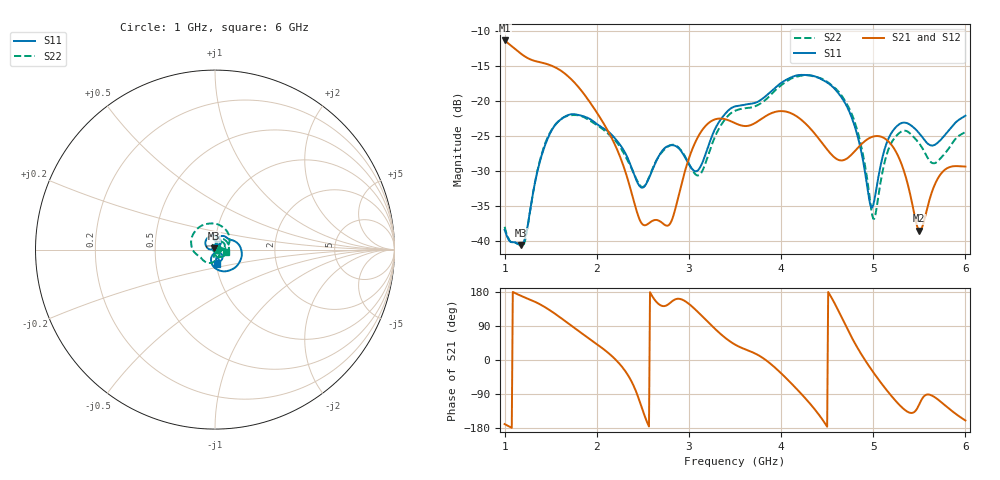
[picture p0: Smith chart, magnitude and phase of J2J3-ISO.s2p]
!Agilent Technologies,E8364B,MY43040528,A.07.50.67
!Agilent E8364B: A.07.50.67
!Date: Sunday, March 01, 2026 20:26:27
!Correction: S11(Full 2 Port(1,2))
!S21(Full 2 Port(1,2))
!S12(Full 2 Port(1,2))
!S22(Full 2 Port(1,2))
!S2P File: Measurements: S11, S21, S12, S22:
# Hz S  dB  R 50
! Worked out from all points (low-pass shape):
!   451 points, 1 GHz to 6 GHz, reference 50 ohm
!   highest |S21| = -11.35 dB at 1 GHz (marker M1); lowest = -38.5 dB at 5.5 GHz (marker M2)
!   |S21| within 3 dB of the highest: start of sweep to 1.349 GHz
!   lowest |S11| = -40.6 dB at 1.178 GHz (marker M3), VSWR 1.02, Z = 49.4 + j0.698 ohm
!   |S11| at or under -10 dB: start of sweep to end of sweep
!   |S22| runs from -40.7 to -16.3 dB; largest |S21 - S12| = 0.00066
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1e9  -38.38 74.1  -11.35 -169.1  -11.37 -169.1  -37.95 16.8
1.177778e9  -40.56 131.1  -13.24 169.3  -13.26 169.2  -40.68 67.7
1.477778e9  -25.04 155.8  -14.79 133.3  -14.80 133.3  -24.88 86.5
1.844444e9  -22.13 91.3  -18.70 69.1  -18.72 69.1  -22.21 4.8
2.211111e9  -25.54 51.8  -26.63 -0.7  -26.65 -0.7  -25.81 -52.4
2.477778e9  -32.30 57.9  -37.27 -117.9  -37.29 -117.9  -32.17 -58.9
2.666667e9  -28.02 81.5  -37.04 148.7  -37.05 148.6  -28.03 -48.9
2.811111e9  -26.30 64.5  -37.11 153.7  -37.13 153.7  -26.26 -75.5
3.111111e9  -29.67 74.7  -24.82 123.5  -24.84 123.5  -30.57 -89.1
3.311111e9  -23.31 78.2  -22.53 75.8  -22.55 75.8  -24.30 -88.6
3.5e9  -20.76 53.5  -23.15 40.7  -23.17 40.7  -21.39 -122.4
4.022222e9  -17.22 10.0  -21.44 -40.1  -21.46 -40.1  -17.54 171.0
4.344444e9  -16.39 -38.3  -24.33 -124.0  -24.35 -123.9  -16.44 109.0
4.6e9  -18.52 -78.4  -28.25 140.6  -28.28 140.6  -18.32 56.1
4.755556e9  -21.98 -103.2  -27.76 64.6  -27.78 64.7  -21.50 23.0
4.877778e9  -27.71 -115.8  -26.08 12.4  -26.11 12.5  -26.95 0.8
5e9  -34.87 -58.2  -25.06 -32.2  -25.09 -32.2  -36.80 33.9
5.166667e9  -25.31 -39.4  -25.78 -85.9  -25.81 -85.9  -26.84 69.1
5.333333e9  -23.08 -65.2  -29.99 -129.8  -30.02 -129.8  -24.23 33.9
5.5e9  -24.62 -83.3  -38.52 -116.7  -38.56 -116.7  -26.08 4.2
5.733333e9  -25.53 -69.9  -30.41 -110.4  -30.43 -110.4  -28.13 10.9
6e9  -22.09 -80.6  -29.35 -159.5  -29.38 -159.6  -24.39 -12.6
